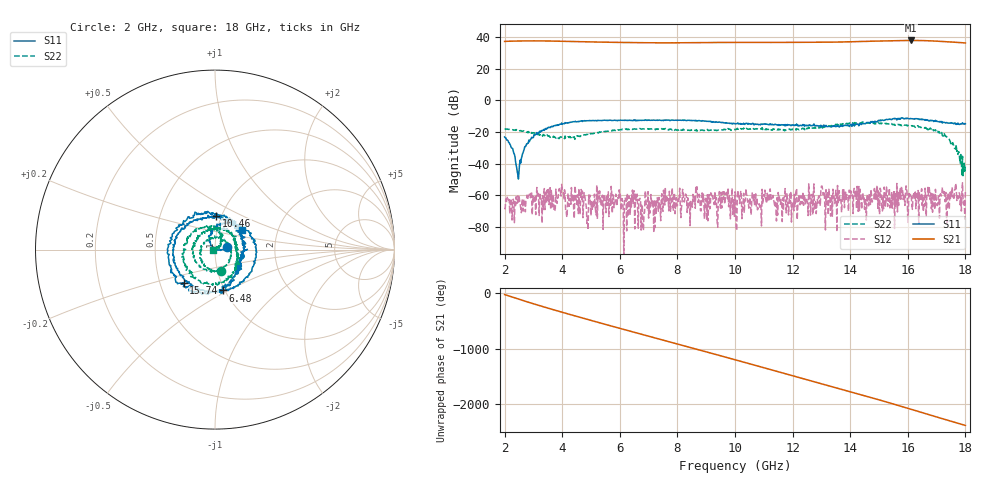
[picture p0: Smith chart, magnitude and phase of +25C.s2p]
!Agilent Technologies,E8361C,US49010292,A.09.42.06
!Agilent E8361C: A.09.42.06
!Date: Wednesday, June 03, 2026 22:43:17
!Correction: S11(Full 2 Port(1,2))
!S21(Full 2 Port(1,2))
!S12(Full 2 Port(1,2))
!S22(Full 2 Port(1,2))
!S2P File: Measurements: S11, S21, S12, S22:
# Hz S  dB  R 50
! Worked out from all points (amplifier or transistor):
!   801 points, 2 GHz to 18 GHz, reference 50 ohm
!   highest |S21| = 37.9 dB at 16.1 GHz (marker M1)
!   |S21| within 3 dB of that: start of sweep to end of sweep
!   unconditionally stable (mu >= 1): start of sweep to end of sweep
!   at 4.66 GHz: K = 4.30, MAG = 37.4 dB, |S12| = -56.3 dB
!   at 10 GHz: K = 5.41, MAG = 36.9 dB, |S12| = -57.7 dB
!   at 18 GHz: K = 5.24, MAG = 36.5 dB, |S12| = -57.0 dB
!   S11 on the Smith chart (normalised r, x): 2 GHz: 1.15, +0.03; 6.48 GHz: 0.98, -0.47; 10.46 GHz: 0.94, +0.37; 15.74 GHz: 0.66, -0.26; 18 GHz: 1.31, +0.29
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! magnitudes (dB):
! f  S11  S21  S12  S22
! 2 GHz  -23.1  37.3  -68.1  -18.1
! 2.48 GHz  -49.7  37.6  -64.7  -19.0
! 3.1 GHz  -21.1  37.6  -61.3  -21.4
! 3.96 GHz  -15.0  37.4  -60.4  -23.0
! 4.2 GHz  -14.3  37.3  -58.6  -22.9
! 4.68 GHz  -12.8  37.1  -62.5  -21.8
! 6.48 GHz  -12.7  36.6  -58.0  -18.0
! 6.78 GHz  -12.5  36.5  -65.7  -18.0
! 7.34 GHz  -12.5  36.4  -70.0  -18.1
! 8.24 GHz  -12.5  36.4  -64.1  -18.5
! 8.42 GHz  -12.6  36.5  -64.4  -19.0
! 8.68 GHz  -12.9  36.5  -54.6  -19.4
! 9.46 GHz  -13.6  36.6  -57.6  -18.8
! 9.68 GHz  -14.4  36.7  -58.5  -18.3
! 10 GHz  -14.8  36.7  -57.7  -18.5
! 10.46 GHz  -14.5  36.7  -63.6  -18.2
! 12.68 GHz  -15.8  36.8  -59.3  -17.4
! 15.34 GHz  -11.8  37.7  -63.4  -14.8
! 15.74 GHz  -11.9  37.9  -55.2  -15.8
! 16.1 GHz  -11.5  37.9  -58.9  -16.0
! 17.34 GHz  -14.0  37.1  -72.2  -23.0
! 18 GHz  -14.7  36.3  -57.0  -41.3
